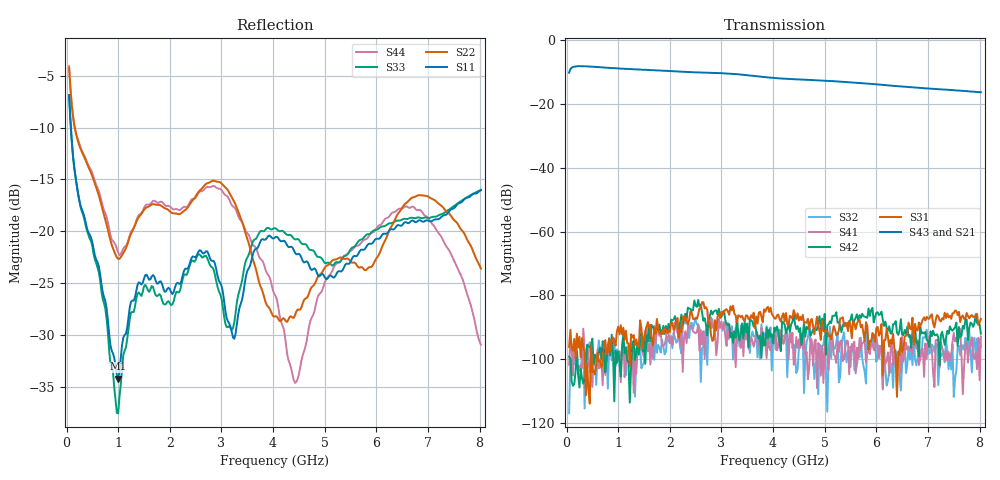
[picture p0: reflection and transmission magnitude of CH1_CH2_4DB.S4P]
!Agilent Technologies,E5071C,MY46316741,A.11.02
!Date: Thu May 28 14:26:22 2026
!Data & Calibration Information:
!1:CH1 INPUT 2:CH1 OUTPUT 3:CH2 INPUT 4:CH2 OUTPUT
!Freq	S11:SOLT4(ON)	S12:SOLT4(ON)	S13:SOLT4(ON)	S14:SOLT4(ON)
!	S21:SOLT4(ON)	S22:SOLT4(ON)	S23:SOLT4(ON)	S24:SOLT4(ON)
!	S31:SOLT4(ON)	S32:SOLT4(ON)	S33:SOLT4(ON)	S34:SOLT4(ON)
!	S41:SOLT4(ON)	S42:SOLT4(ON)	S43:SOLT4(ON)	S44:SOLT4(ON)
!PortZ  Port1:50+j0  Port2:50+j0  Port3:50+j0  Port4:50+j0
!Above PortZ is port z conversion or system Z0 setting when saving the data.
!When reading, reference impedance value at option line is always used.
# Hz S dB R 50
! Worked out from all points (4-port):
!   320 points, 50 MHz to 8.025 GHz, reference 50 ohm
!   strongest paths, dB at 50 MHz, 2.05 GHz, 4.05 GHz, 6.05 GHz, 8.025 GHz:
!     S43: -10.2, -9.7, -11.9, -13.9, -16.3
!     S21: -10.3, -9.8, -12.0, -13.9, -16.4
!     S31: -96.2, -88.5, -87.3, -92.6, -87.4
!     S42: -99.2, -87.8, -91.2, -86.1, -92.0
!     S41: -101.7, -95.6, -91.7, -99.7, -92.9
!     S32: -117.0, -96.6, -97.0, -95.7, -96.1
!   lowest |S11| = -34.2 dB at 1 GHz (marker M1), VSWR 1.04, Z = 48.7 - j1.45 ohm
!   |S11| at or under -10 dB: 84.38 MHz to end of sweep
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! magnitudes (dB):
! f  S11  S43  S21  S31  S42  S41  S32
! 50 MHz  -6.9  -10.2  -10.3  -96.2  -99.2  -101.7  -117.0
! 1 GHz  -34.2  -8.8  -9.0  -89.8  -97.5  -98.0  -98.7
! 1.5 GHz  -24.6  -9.3  -9.4  -93.2  -93.7  -99.6  -101.1
! 2.975 GHz  -25.0  -10.3  -10.5  -87.1  -86.2  -90.2  -88.6
! 4.425 GHz  -22.1  -12.3  -12.3  -86.1  -88.9  -99.4  -98.9
! 6.7 GHz  -19.0  -14.8  -14.9  -87.0  -91.1  -98.3  -101.8
! 8.025 GHz  -16.0  -16.3  -16.4  -87.4  -92.0  -92.9  -96.1
